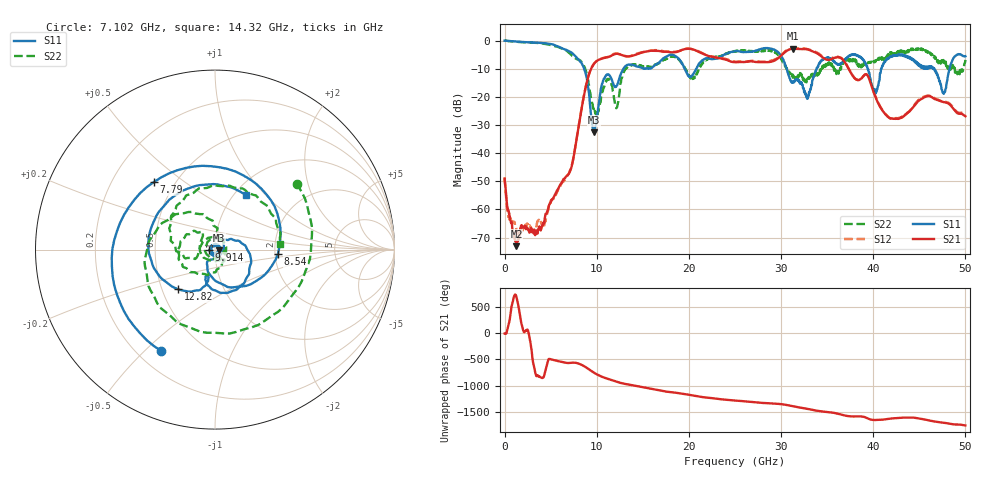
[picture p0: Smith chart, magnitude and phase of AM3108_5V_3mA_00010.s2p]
# Hz S DB R 50.0
!freq dBS11 angS11 dBS21 angS21 dBS12 angS12 dBS22 angS22
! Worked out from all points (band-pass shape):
!   1601 points, 10 MHz to 50 GHz, reference 50 ohm
!   highest |S21| = -2.83 dB at 31.28 GHz (marker M1); lowest = -73.0 dB at 1.291 GHz (marker M2)
!   |S21| within 3 dB of the highest: 11.24 GHz to 22.72 GHz (11.48 GHz wide, 67.6 % of centre); 29.81 GHz to 34.47 GHz (4.664 GHz wide, 14.5 % of centre)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
!   lowest |S11| = -32.5 dB at 9.664 GHz (marker M3), VSWR 1.05, Z = 52.4 - j0.347 ohm
!   |S11| at or under -10 dB: 8.65 GHz to 12.89 GHz (4.243 GHz wide, 39.4 % of centre); 30.62 GHz to 33.84 GHz (3.223 GHz wide, 10 % of centre); 46.63 GHz to 48.28 GHz (1.655 GHz wide, 3.49 % of centre)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
!   |S22| runs from -26.8 to 0.1 dB; largest |S21 - S12| = 0.023
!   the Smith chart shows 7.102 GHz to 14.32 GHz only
!   S11 on the Smith chart (normalised r, x): 7.102 GHz: 0.30, -0.56; 7.79 GHz: 0.38, +0.39; 8.54 GHz: 2.08, -0.12; 9.914 GHz: 0.94, -0.00; 12.82 GHz: 0.60, -0.29; 14.32 GHz: 1.14, +0.78
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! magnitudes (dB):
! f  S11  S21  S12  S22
! 10 MHz  0.0  -49.0  -48.7  0.1
! 1.291 GHz  -0.3  -73.0  -68.4  -0.4
! 4.259 GHz  -0.9  -65.0  -66.4  -1.1
! 7.102 GHz  -3.9  -46.4  -46.2  -4.6
! 7.79 GHz  -5.9  -35.6  -35.5  -6.4
! 8.352 GHz  -7.9  -24.2  -24.2  -7.5
! 8.54 GHz  -9.1  -20.9  -20.7  -8.5
! 9.664 GHz  -32.5  -8.4  -8.3  -24.0
! 9.914 GHz  -30.0  -7.4  -7.5  -25.3
! 10.82 GHz  -13.4  -6.1  -6.0  -16.2
! 12.16 GHz  -16.1  -4.6  -4.6  -23.9
! 12.82 GHz  -10.4  -5.2  -5.2  -12.0
! 14.32 GHz  -9.1  -4.9  -4.6  -8.8
! 16.69 GHz  -7.9  -3.6  -3.3  -8.2
! 25 GHz  -3.7  -7.6  -7.4  -3.8
! 31.28 GHz  -14.9  -2.8  -2.8  -13.1
! 33.35 GHz  -15.6  -3.7  -3.5  -12.7
! 38 GHz  -4.8  -13.4  -13.4  -6.6
! 40.22 GHz  -18.9  -19.8  -19.6  -7.6
! 41.69 GHz  -6.1  -27.3  -27.3  -5.2
! 47.66 GHz  -18.9  -21.8  -21.7  -7.7
! 50 GHz  -5.5  -26.9  -26.5  -6.8
